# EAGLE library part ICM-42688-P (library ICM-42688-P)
IMU (Inertial Measurement Unit), 6-Axis, Accelerometer, Gyroscope Source: Datasheet
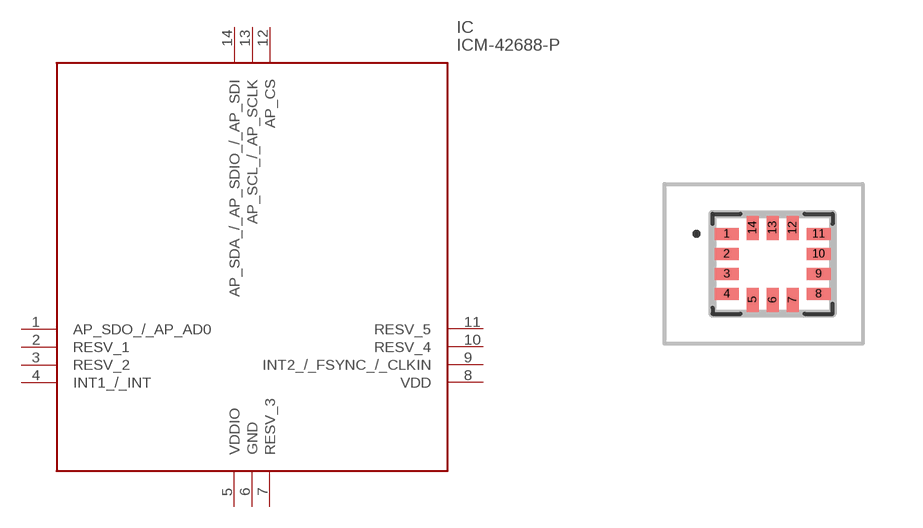
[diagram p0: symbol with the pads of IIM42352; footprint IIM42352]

Designator prefix IC

## ICM-42688-P (Arrow_Part_Number: ICM-42688-P; Arrow_Price-Stock: https://www.arrow.com/en/products/icm-42688-p/invensense?utm_currency=USD&region=nac; Description: IMU (Inertial Measurement Unit), 6-Axis, Accelerometer, Gyroscope; Height: mm; Manufacturer_Name: TDK; Manufacturer_Part_Number: ICM-42688-P; Mouser_Part_Number: 410-ICM-42688-P; Mouser_Price-Stock: https://www.mouser.co.uk/ProductDetail/TDK-InvenSense/ICM-42688-P?qs=OlC7AqGiEDk8QrNAV728zw%3D%3D)  [IIM42352]
1  AP_SDO_/_AP_AD0
2  RESV_1
3  RESV_2
4  INT1_/_INT
5  VDDIO
6  GND
7  RESV_3
8  VDD
9  INT2_/_FSYNC_/_CLKIN
10  RESV_4
11  RESV_5
12  AP_CS
13  AP_SCL_/_AP_SCLK
14  AP_SDA_/_AP_SDIO_/_AP_SDI

## Footprint IIM42352 (pad centres in mm)
14 Lead LGA (2.5x3x0.91)_1
smd 0.6 x 0.3: 1 -1.15,0.75; 2 -1.15,0.25; 3 -1.15,-0.25; 4 -1.15,-0.75; 8 1.15,-0.75; 9 1.15,-0.25; 10 1.15,0.25; 11 1.15,0.75
smd 0.3 x 0.6: 5 -0.5,-0.9; 6 0,-0.9; 7 0.5,-0.9; 12 0.5,0.9; 13 0,0.9; 14 -0.5,0.9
